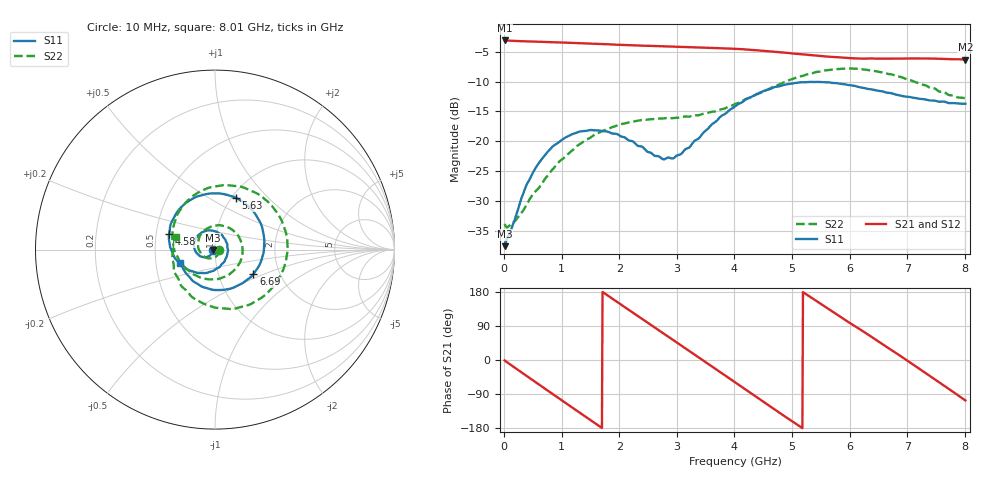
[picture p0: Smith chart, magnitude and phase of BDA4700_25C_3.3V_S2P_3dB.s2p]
!Agilent Technologies,E5071B,MY42404982,A.09.10
!Date: Mon Oct 20 18:04:14 2025
!Data & Calibration Information:
!Freq	S11:SOLT2(ON)	S21:SOLT2(ON)	S12:SOLT2(ON)	S22:SOLT2(ON)
# Hz S RI R 50
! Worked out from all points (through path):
!   801 points, 10 MHz to 8.01 GHz, reference 50 ohm
!   highest |S21| = -3.12 dB at 10 MHz (marker M1); lowest = -6.3 dB at 8.01 GHz (marker M2)
!   group delay of S21, straight-line fit = 286 ps
!   lowest |S11| = -37.6 dB at 10 MHz (marker M3), VSWR 1.03, Z = 48.7 - j0.158 ohm
!   |S11| at or under -10 dB: start of sweep to end of sweep
!   |S22| runs from -34.5 to -7.8 dB; largest |S21 - S12| = 0.0079
!   S11 on the Smith chart (normalised r, x): 10 MHz: 0.97, -0.00; 4.58 GHz: 0.59, +0.11; 5.63 GHz: 1.05, +0.67; 6.69 GHz: 1.47, -0.43; 8.01 GHz: 0.67, -0.10
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1e7  -0.0131 -0.00162  0.6984 -0.0146  0.6983 -0.0155  0.0201 -0.0018
3.3e8  -0.0231 -0.0279  0.5605 -0.3989  0.56 -0.3991  0.018 -0.0189
7.2e8  -0.065 -0.0422  0.156 -0.6601  0.1564 -0.66  -0.0117 -0.0475
1.02e9  -0.1019 -0.0197  -0.2097 -0.6371  -0.2097 -0.6374  -0.0589 -0.0398
1.35e9  -0.1167 0.0318  -0.5273 -0.3998  -0.5274 -0.3999  -0.0946 0.0202
1.64e9  -0.0943 0.0794  -0.6488 -0.0783  -0.6485 -0.0783  -0.0747 0.0905
1.93e9  -0.0464 0.1057  -0.5918 0.255  -0.592 0.2555  -0.0011 0.1334
2.32e9  0.0256 0.0879  -0.2816 0.5681  -0.2815 0.5681  0.1131 0.096
2.68e9  0.0674 0.032  0.1171 0.6155  0.1162 0.6148  0.1535 -0.0179
3.36e9  0.0159 -0.1025  0.6035 0.0958  0.6045 0.0958  -0.000383 -0.1646
3.67e9  -0.0636 -0.1302  0.5549 -0.2376  0.5548 -0.2393  -0.102 -0.1458
4.01e9  -0.1666 -0.1025  0.3085 -0.508  0.3096 -0.5067  -0.1909 -0.0736
4.58e9  -0.2555 0.0869  -0.268 -0.5007  -0.2679 -0.5013  -0.2251 0.1508
4.97e9  -0.182 0.2422  -0.5076 -0.201  -0.5079 -0.2029  -0.1082 0.3089
5.35e9  -0.0175 0.3129  -0.5022 0.1546  -0.503 0.1521  0.1068 0.3549
5.63e9  0.1177 0.2881  -0.3615 0.3616  -0.3612 0.362  0.2695 0.2884
6.14e9  0.2673 0.1012  0.0471 0.4914  0.0509 0.4921  0.4038 -0.0104
6.68e9  0.2164 -0.1332  0.4219 0.2514  0.4228 0.251  0.2231 -0.2895
6.69e9  0.2139 -0.1365  0.4264 0.2444  0.427 0.2436  0.2172 -0.2928
7.25e9  0.00852 -0.2257  0.4388 -0.2267  0.4383 -0.2271  -0.0954 -0.2834
7.64e9  -0.1238 -0.1752  0.1836 -0.4522  0.1835 -0.4531  -0.2281 -0.1221
8.01e9  -0.1929 -0.0728  -0.1388 -0.4628  -0.1376 -0.4632  -0.2187 0.0684
